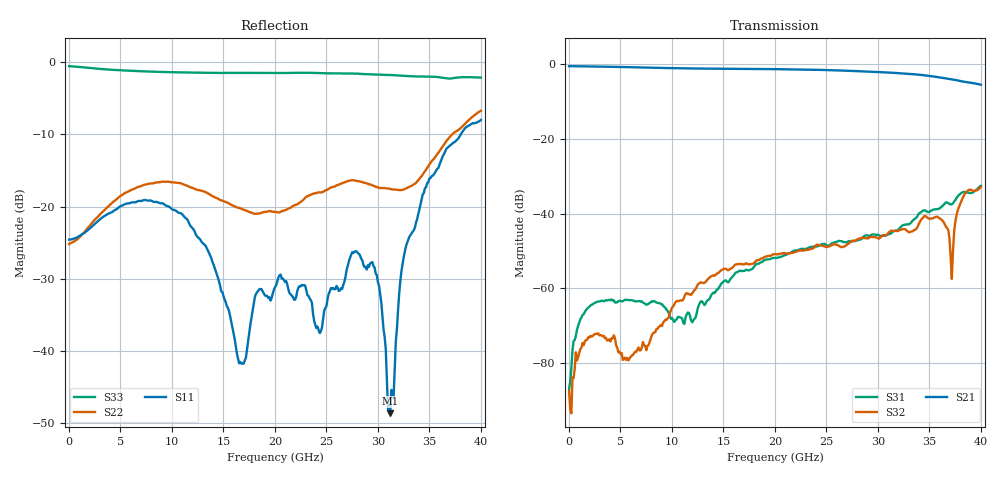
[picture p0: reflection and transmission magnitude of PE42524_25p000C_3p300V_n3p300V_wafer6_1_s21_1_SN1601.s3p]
!Agilent Technologies,N5224A,MY51441010,A.09.90.07
!Agilent N5224A: A.09.90.07
!Date: Wednesday, September 10, 2014 09:34:32
!Correction: S11(Full 3 Port(1,2,3))
!S12(Full 3 Port(1,2,3))
!S13(Full 3 Port(1,2,3))
!S21(Full 3 Port(1,2,3))
!S22(Full 3 Port(1,2,3))
!S23(Full 3 Port(1,2,3))
!S31(Full 3 Port(1,2,3))
!S32(Full 3 Port(1,2,3))
!S33(Full 3 Port(1,2,3))
!S3P File: Measurements: <S11,S12,S13>,
!<S21,S22,S23>,
!<S31,S32,S33>:
# Hz S  dB  R 50
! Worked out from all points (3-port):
!   369 points, 10 MHz to 40.02 GHz, reference 50 ohm
!   strongest paths, dB at 10 MHz, 10.01 GHz, 20.02 GHz, 30.02 GHz, 40.02 GHz:
!     S21: -0.6, -1.1, -1.4, -2.1, -5.5
!     S32: -87.4, -65.1, -50.8, -46.5, -32.8
!     S31: -86.8, -67.9, -51.8, -45.6, -32.6
!   lowest |S11| = -48.7 dB at 31.21 GHz (marker M1), VSWR 1.01, Z = 49.8 - j0.297 ohm
!   |S11| at or under -10 dB: start of sweep to 38.05 GHz
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1e7  -24.59 -0.9  -0.58 -0.2  -95.44 107.0
     -0.58 -0.1  -25.20 -0.4  -94.26 -112.2
     -86.85 88.1  -87.42 -6.2  -0.52 179.9
7.729475e9  -19.17 -150.3  -0.97 -100.7  -64.17 -7.9
            -0.97 -100.8  -16.85 -168.4  -75.10 160.0
            -64.13 -8.2  -75.15 161.8  -1.26 120.9
1.39268e10  -27.65 142.5  -1.25 -179.9  -61.42 31.2
            -1.25 -179.9  -18.55 106.9  -56.53 53.8
            -61.41 31.4  -56.57 53.9  -1.45 74.5
2.00154e10  -31.18 -145.1  -1.38 100.3  -51.84 -30.8
            -1.38 100.2  -20.75 38.2  -50.86 -48.0
            -51.84 -31.1  -50.82 -48.0  -1.45 25.4
2.947448e10  -27.70 -109.0  -2.09 -30.7  -45.58 -133.3
             -2.08 -30.8  -17.04 -89.1  -46.25 169.9
             -45.57 -133.3  -46.25 170.0  -1.67 -58.6
3.121408e10  -48.68 -125.9  -2.31 -55.9  -45.39 -144.6
             -2.30 -56.0  -17.56 -99.2  -44.72 152.8
             -45.41 -144.7  -44.72 152.9  -1.75 -73.9
3.621542e10  -13.39 -42.7  -3.68 -132.2  -38.13 163.2
             -3.67 -132.3  -11.85 -108.1  -41.59 78.3
             -38.14 163.0  -41.59 78.2  -2.11 -119.6
3.719395e10  -11.33 -54.8  -4.09 -147.2  -37.49 150.7
             -4.09 -147.3  -10.04 -118.3  -57.53 110.5
             -37.49 150.4  -57.47 110.5  -2.21 -127.4
3.773758e10  -10.69 -62.6  -4.39 -155.8  -35.48 148.7
             -4.38 -155.9  -9.46 -125.6  -39.47 137.6
             -35.48 148.5  -39.47 137.5  -2.11 -132.7
4.00208e10  -7.99 -90.0  -5.55 168.8  -32.56 116.8
            -5.54 168.6  -6.70 -157.3  -32.84 77.9
            -32.55 116.6  -32.84 77.9  -2.11 -156.5
